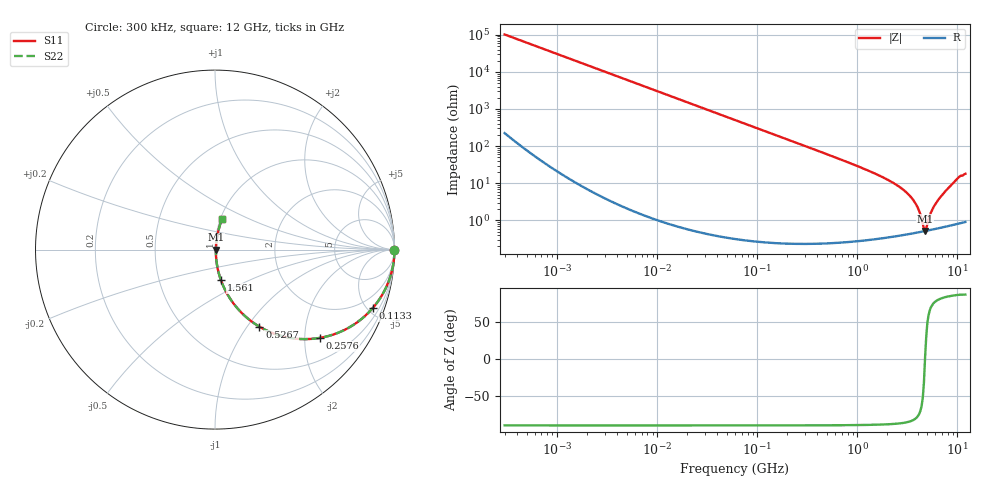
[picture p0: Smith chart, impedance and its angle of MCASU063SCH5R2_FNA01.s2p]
! MCASU063SCH5R2_FNA01  S-PARAMETER MODEL  ( General Type )
! Model Generated by TAIYO YUDEN Corporation (http://www.ty-top.com)
! Version 1.0
! TAIYO YUDEN Control No. 130801
! Copyright(c) 2013 TAIYO YUDEN CO.,LTD. All Rights Reserved.
! Product Description (link to TY-COMPAS)
! https://ds.yuden.co.jp/TYCOMPAS/or/detail?pn=MCASU063SCH5R2DFNA01&u=M
! Products Name : Multilayer Ceramic Capacitors
! Characteristics :
!  Capacitance : 5.2 pF , Rated Voltage : 50V , TCC : CH / C0H
!  Case Size : 0.6 x 0.3 / 0.024 x 0.012 [mm/inch] , Thickness : 0.3 / 0.012 [mm/inch]
!  (Conditions: Temperature = 25 degC , DC Bias Current/Voltage = 0A / 0V)
! External Node Assignments :
!  1  o---| |---o  2
! GND o---------o GND
! Frequency Range : 0.3MHz  -  12000MHz  [ 401 STEP ]
# MHz S RI R 50
! Freq[MHz].  S11 Real  S11 Imag  S21 Real  S21 Imag  S12 Real  S12 Imag  S22 Real  S22 Imag
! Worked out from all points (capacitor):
!   401 points, 300 kHz to 12 GHz, reference 50 ohm
!   read as one part in series: C = 5.21 pF near 316.3 kHz
!   lowest |Z| = 519 mohm at 4.748 GHz (marker M1)
!   series resonance near 4.741 GHz, so ESL is about 220 pH
!   S11 on the Smith chart (normalised r, x): 300 kHz: open; 113.3 MHz: 1.01, -5.39; 257.6 MHz: 1.00, -2.36; 526.7 MHz: 1.00, -1.15; 1.561 GHz: 1.01, -0.35; 12 GHz: 1.02, +0.36
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0.3  1 -0.000982  3.14e-06 0.000982  3.14e-06 0.000982  1 -0.000982
1.769972  1 -0.0058  3.64e-05 0.0058  3.64e-05 0.0058  1 -0.0058
10.44266  0.9988 -0.0342  0.00118 0.0342  0.00118 0.0342  0.9988 -0.0342
27.82928  0.9917 -0.0904  0.00827 0.0904  0.00827 0.0904  0.9917 -0.0904
60  0.9627 -0.1892  0.0373 0.1892  0.0373 0.1892  0.9627 -0.1892
113.3117  0.8786 -0.3261  0.1214 0.3261  0.1214 0.3261  0.8786 -0.3261
257.5933  0.5827 -0.4921  0.4173 0.4921  0.4173 0.4921  0.5827 -0.4921
353.9943  0.4241 -0.4928  0.5759 0.4928  0.5759 0.4928  0.4241 -0.4928
526.7124  0.2479 -0.4297  0.7521 0.4297  0.7521 0.4297  0.2479 -0.4297
871.3074  0.1048 -0.3024  0.8952 0.3024  0.8952 0.3024  0.1048 -0.3024
1560.575  0.0324 -0.1683  0.9676 0.1683  0.9676 0.1683  0.0324 -0.1683
2088.533  0.0171 -0.1154  0.9829 0.1154  0.9829 0.1154  0.0171 -0.1154
2870.14  0.00849 -0.0666  0.9915 0.0666  0.9915 0.0666  0.00849 -0.0666
3547.679  0.00586 -0.0375  0.9941 0.0375  0.9941 0.0375  0.00586 -0.0375
4050.141  0.00516 -0.0202  0.9948 0.0202  0.9948 0.0202  0.00516 -0.0202
4502.883  0.00506 -0.00657  0.9949 0.00657  0.9949 0.00657  0.00506 -0.00657
4747.894  0.00516 0.000179  0.9948 -0.000179  0.9948 -0.000179  0.00516 0.000179
5006.236  0.00535 0.00612  0.9946 -0.00612  0.9946 -0.00612  0.00535 0.00612
5715.274  0.00616 0.0209  0.9938 -0.0209  0.9938 -0.0209  0.00616 0.0209
6524.734  0.00754 0.0368  0.9925 -0.0368  0.9925 -0.0368  0.00754 0.0368
9968.853  0.025 0.1287  0.975 -0.1287  0.975 -0.1287  0.025 0.1287
12000  0.0397 0.1717  0.9603 -0.1717  0.9603 -0.1717  0.0397 0.1717
